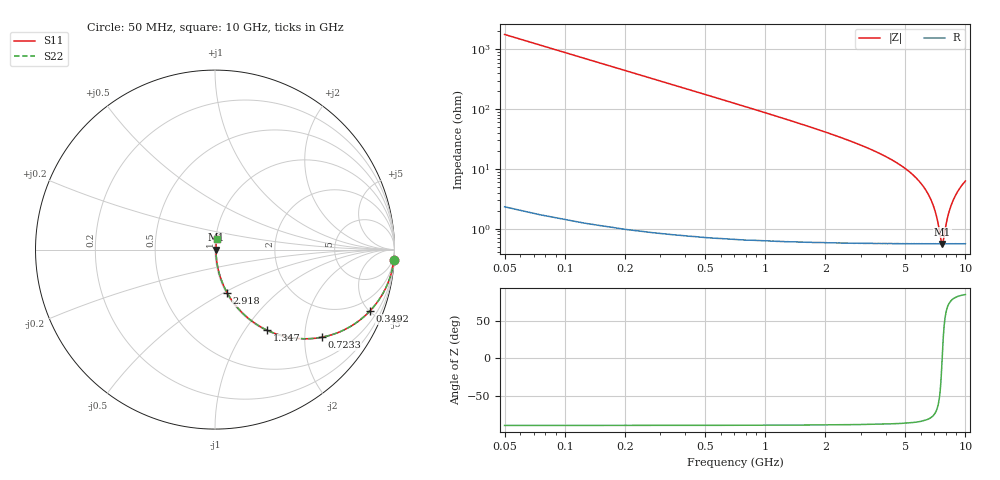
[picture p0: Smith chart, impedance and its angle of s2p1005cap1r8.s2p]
!	AVX	Thin	Film	Operation
!	Date:	March 2012
!	Description: Ultra-Miniature 01005 Size ACCU - P® Thin Film RF / Microwave Capacitor
!	Part Number:  C005YK1R8ABSTR
!	Serial	Measurements
#	MHz	S	db	R	50
!	S11	S21	S12	S22
!	dB	Phase	dB	Phase	dB	Phase	dB	Phase
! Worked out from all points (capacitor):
!   400 points, 50 MHz to 10 GHz, reference 50 ohm
!   read as one part in series: C = 1.8 pF near 99.88 MHz
!   lowest |Z| = 556 mohm at 7.656 GHz (marker M1)
!   series resonance near 7.657 GHz, so ESL is about 240 pH
!   S11 on the Smith chart (normalised r, x): 50 MHz: 1, -35; 349.2 MHz: 1.02, -5.05; 723.3 MHz: 1.01, -2.42; 1.347 GHz: 1.01, -1.27; 2.918 GHz: 1.01, -0.52; 10 GHz: 1.01, +0.12
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50  -0.01 -3.2  -24.97 86.7  -24.97 86.7  -0.01 -3.2
99.875  -0.06 -6.4  -19.00 83.5  -19.00 83.5  -0.06 -6.4
149.749  -0.13 -9.6  -15.55 80.3  -15.55 80.3  -0.13 -9.6
224.561  -0.28 -14.3  -12.17 75.6  -12.17 75.6  -0.28 -14.3
349.248  -0.64 -21.6  -8.69 68.3  -8.69 68.3  -0.64 -21.6
523.81  -1.33 -30.7  -5.84 59.1  -5.84 59.1  -1.33 -30.7
723.308  -2.28 -39.4  -3.95 50.3  -3.95 50.3  -2.28 -39.4
1346.742  -5.44 -57.1  -1.51 32.3  -1.51 32.3  -5.44 -57.1
1720.802  -7.20 -63.4  -0.97 25.9  -0.97 25.9  -7.20 -63.4
2917.794  -12.06 -74.3  -0.33 14.4  -0.33 14.4  -12.06 -74.3
3366.667  -13.71 -76.6  -0.24 11.9  -0.24 11.9  -13.71 -76.6
5037.469  -20.11 -81.1  -0.09 5.7  -0.09 5.7  -20.11 -81.1
6010.025  -24.98 -81.1  -0.06 3.2  -0.06 3.2  -24.98 -81.1
6708.271  -30.18 -77.9  -0.05 1.7  -0.05 1.7  -30.18 -77.9
7157.143  -35.66 -69.5  -0.05 0.9  -0.05 0.9  -35.66 -69.5
7556.14  -43.98 -28.7  -0.05 0.2  -0.05 0.2  -43.98 -28.7
7655.89  -45.13 -0.4  -0.05 0.0  -0.05 0.0  -45.13 -0.4
7755.639  -44.06 27.7  -0.05 -0.2  -0.05 -0.2  -44.06 27.7
8079.825  -37.38 65.1  -0.05 -0.7  -0.05 -0.7  -37.38 65.1
8354.135  -33.65 73.4  -0.05 -1.1  -0.05 -1.1  -33.65 73.4
9027.444  -28.32 79.5  -0.06 -2.2  -0.06 -2.2  -28.32 79.5
10000  -24.13 81.3  -0.07 -3.5  -0.07 -3.5  -24.13 81.3
